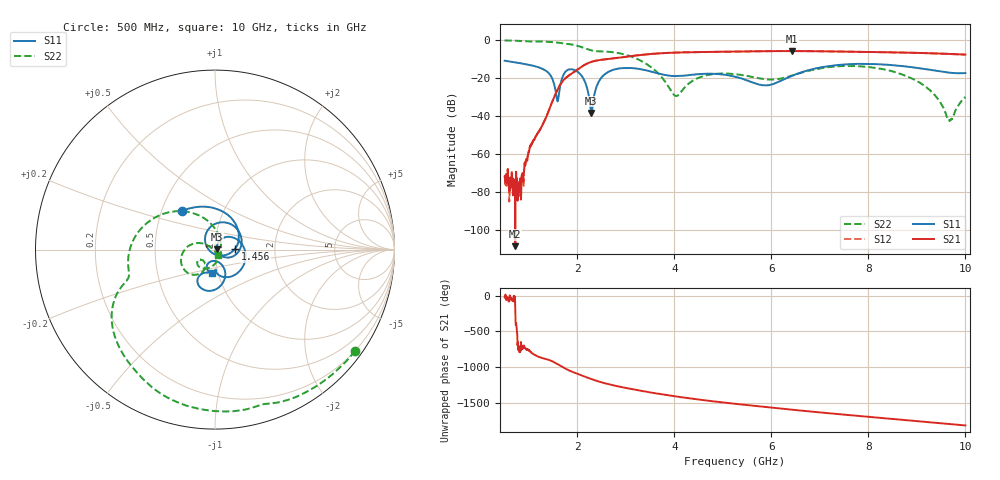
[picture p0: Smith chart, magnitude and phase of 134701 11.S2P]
!  2-Port S-parameters saved by WinCal
! VAR MeasName=S-Parameters (CALIBRATED_DATA) read from VNA (N5242A)
! VAR MeasDate=2013-7-3 16:28:55
! VAR NAME=134701 11
! VAR FILENAME=134701 11.S2P
! VAR DATE=2013-7-3 16:28:55
! VAR PHYS_PORTS=1,2
# Hz S MA R 50
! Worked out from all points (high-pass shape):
!   1601 points, 500 MHz to 10 GHz, reference 50 ohm
!   highest |S21| = -5.90 dB at 6.426 GHz (marker M1); lowest = -108.5 dB at 719.7 MHz (marker M2)
!   |S21| within 3 dB of the highest: 3.013 GHz to end of sweep
!   lowest |S11| = -38.4 dB at 2.287 GHz (marker M3), VSWR 1.02, Z = 51.2 + j0.104 ohm
!   |S11| at or under -10 dB: start of sweep to end of sweep
!   |S22| runs from -42.6 to -0.3 dB; largest |S21 - S12| = 0.0023
!   S11 on the Smith chart (normalised r, x): 500 MHz: 0.64, +0.30; 1.456 GHz: 1.25, +0.01; 10 GHz: 0.94, -0.25
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5e8  0.2826 130.1  0.0002494 -19.0  0.000174 -0.2  0.9631 -35.9
7.196875e8  0.2546 110.3  3.739e-06 172.5  0.0001106 -68.7  0.9493 -51.5
8.0875e8  0.2439 101.9  0.0001418 -72.0  9.912e-05 -32.4  0.9419 -57.9
1.04625e9  0.2142 76.6  0.001656 -71.2  0.00164 -71.4  0.9024 -73.7
1.455938e9  0.1112 1.7  0.01947 170.4  0.01948 170.5  0.8763 -103.5
1.586562e9  0.02461 -106.6  0.0476 126.7  0.04752 126.6  0.8466 -113.7
1.7825e9  0.1563 76.6  0.1049 49.9  0.1047 49.8  0.7875 -128.4
2.085312e9  0.1146 -16.4  0.1962 -34.7  0.1958 -34.8  0.6453 -151.7
2.287188e9  0.01196 4.9  0.2635 -86.1  0.2625 -86.1  0.5293 -160.2
2.4475e9  0.08227 53.7  0.2929 -122.3  0.2923 -122.2  0.4979 -164.3
2.66125e9  0.1481 15.0  0.3167 -161.3  0.3165 -161.2  0.4831 -175.8
3.670625e9  0.1303 -86.3  0.4396 67.7  0.4393 67.8  0.1295 94.2
4.03875e9  0.1117 -87.8  0.4627 29.4  0.4622 29.3  0.03354 -7.2
4.543438e9  0.1261 -94.0  0.4779 -16.6  0.4777 -16.7  0.1053 -107.6
5.25e9  0.1071 -115.6  0.492 -72.5  0.4921 -72.5  0.1256 -142.1
5.89125e9  0.06365 -92.4  0.5036 -118.5  0.503 -118.6  0.09119 -140.3
6.425625e9  0.1125 -64.3  0.5072 -155.3  0.5069 -155.3  0.1151 -119.0
6.835312e9  0.1682 -71.0  0.5028 177.6  0.503 177.6  0.1607 -122.7
8.420625e9  0.2197 -114.4  0.4701 79.7  0.4692 79.7  0.1571 175.1
9.222188e9  0.1662 -120.5  0.4455 31.2  0.4462 31.3  0.05295 150.3
9.673438e9  0.1369 -111.2  0.4256 4.2  0.426 4.0  0.007803 -144.3
1e10  0.1339 -96.5  0.4081 -15.7  0.4089 -15.7  0.03138 -63.2
